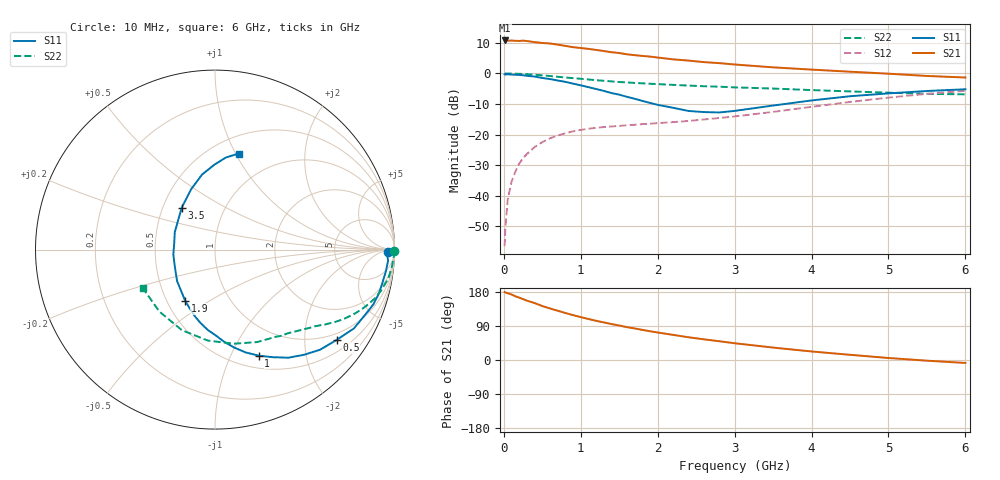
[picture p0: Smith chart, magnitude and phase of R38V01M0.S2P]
! SIEMENS Small Signal Semiconductors
! BFR181
! Si NPN RF Bipolar Junction Transistor in SOT23
! VCE = 8 V  IC = 1 mA
! Common Emitter S-Parameters:  May  1996
# GHz  S  MA  R  50
!  f  S11  S21  S12  S22
! GHz  MAG  ANG  MAG  ANG  MAG  ANG  MAG  ANG
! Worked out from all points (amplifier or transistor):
!   36 points, 10 MHz to 6 GHz, reference 50 ohm
!   highest |S21| = 10.8 dB at 10 MHz (marker M1)
!   |S21| within 3 dB of that: start of sweep to 1.171 GHz
!   unconditionally stable (mu >= 1): 2.077 GHz to 3.717 GHz
!   at 250 MHz: K = 0.15, MSG = 19.2 dB, |S12| = -27.7 dB
!   at 1.4 GHz: K = 0.76, MSG = 12.1 dB, |S12| = -17.3 dB
!   at 6 GHz: K = 0.87, MSG = 2.2 dB, |S12| = -5.7 dB
!   lowest NFmin = 1.30 dB at 450 MHz
!   S11 on the Smith chart (normalised r, x): 10 MHz: 50, -20; 500 MHz: 0.80, -2.82; 1 GHz: 0.64, -1.28; 1.9 GHz: 0.62, -0.40; 3.5 GHz: 0.62, +0.32; 6 GHz: 0.67, +1.03
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0.01  0.9662 -0.8  3.463 179.3  0.0015 89.7  0.9987 -0.4
0.02  0.9593 -1.6  3.448 178.2  0.003 93.4  0.9961 -0.8
0.05  0.9665 -3.7  3.423 176.3  0.0086 88.6  0.9977 -1.8
0.1  0.9594 -7.3  3.454 172.8  0.017 86.9  0.9936 -3.6
0.2  0.9452 -15.0  3.399 164.6  0.0336 80.4  0.9851 -7.2
0.25  0.9337 -19.0  3.437 160.7  0.0412 77.5  0.9804 -9.0
0.3  0.9156 -22.7  3.388 156.6  0.0483 75.7  0.9711 -10.7
0.5  0.8441 -36.6  3.152 142.4  0.0753 66.8  0.9324 -16.8
0.6  0.8088 -43.6  3.087 136.0  0.0871 62.9  0.9073 -19.6
0.7  0.7674 -49.8  2.963 130.0  0.0967 59.8  0.8827 -22.1
0.9  0.6818 -61.6  2.69 118.4  0.1131 54.0  0.8383 -26.2
1  0.6391 -67.6  2.605 113.2  0.1194 51.8  0.817 -28.1
1.1  0.5972 -73.5  2.522 108.2  0.1248 49.9  0.7966 -29.8
1.4  0.4782 -89.5  2.224 94.8  0.1358 46.1  0.741 -34.3
1.6  0.4152 -101.5  2.056 86.7  0.1421 44.9  0.7125 -36.6
1.9  0.33 -120.2  1.887 75.9  0.1506 44.6  0.6787 -40.2
2.2  0.2747 -140.3  1.7 66.3  0.1599 45.6  0.6508 -43.8
2.8  0.2301 170.6  1.475 49.5  0.1867 49.1  0.6077 -52.1
3.5  0.2988 128.3  1.258 32.8  0.2352 51.3  0.5662 -65.5
4.5  0.4243 99.8  1.068 13.7  0.3419 47.4  0.5085 -94.6
5.5  0.5164 83.3  0.91 -1.8  0.4638 35.5  0.4639 -132.0
6  0.5512 76.2  0.858 -7.8  0.5197 27.8  0.4558 -152.1
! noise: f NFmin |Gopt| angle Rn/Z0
0.45  1.3  0.7  18  0.5
0.9  1.4  0.6  39  0.52
1.8  1.85  0.4  81  0.47
